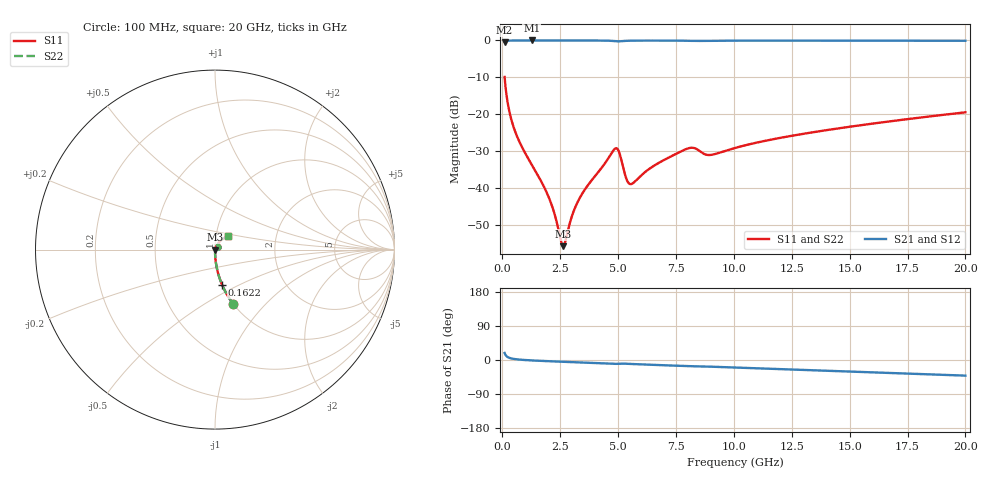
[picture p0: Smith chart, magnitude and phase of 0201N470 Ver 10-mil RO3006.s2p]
# GHz S MA R 50
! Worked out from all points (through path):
!   1601 points, 100 MHz to 20 GHz, reference 50 ohm
!   highest |S21| = -0.01 dB at 1.269 GHz (marker M1); lowest = -0.5 dB at 100 MHz (marker M2)
!   group delay of S21, straight-line fit = 5.97 ps
!   lowest |S11| = -55.8 dB at 2.625 GHz (marker M3), VSWR 1.00, Z = 50.2 - j0.0251 ohm
!   |S11| at or under -10 dB: 101.2 MHz to end of sweep
!   |S22| runs from -55.8 to -9.9 dB; largest |S21 - S12| = 0
!   S11 on the Smith chart (normalised r, x): 100 MHz: 1.00, -0.67; 162.2 MHz: 1.00, -0.41; 20 GHz: 1.14, +0.18
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0.1  0.3195 -71.5  0.9472 18.5  0.9472 18.5  0.3195 -71.5
0.1621875  0.2031 -78.4  0.9787 11.4  0.9787 11.4  0.2031 -78.4
0.3114375  0.1064 -84.2  0.9938 5.5  0.9938 5.5  0.1064 -84.2
0.522875  0.06203 -86.8  0.9975 2.6  0.9975 2.6  0.06203 -86.8
1.269125  0.02071 -88.3  0.9988 -1.1  0.9988 -1.1  0.02071 -88.3
2.04025  0.007008 -82.1  0.9986 -3.3  0.9986 -3.3  0.007008 -82.1
2.53775  0.001883 -37.9  0.9984 -4.5  0.9984 -4.5  0.001883 -37.9
2.624812  0.001617 -8.9  0.9983 -4.7  0.9983 -4.7  0.001617 -8.9
2.724312  0.001891 23.7  0.9983 -5.0  0.9983 -5.0  0.001891 23.7
3.085  0.004843 61.7  0.9981 -5.8  0.9981 -5.8  0.004843 61.7
3.420812  0.008032 68.3  0.9978 -6.6  0.9978 -6.6  0.008032 68.3
4.876  0.03416 38.1  0.9768 -10.2  0.9768 -10.2  0.03416 38.1
5.02525  0.03158 15.4  0.9712 -9.8  0.9712 -9.8  0.03158 15.4
5.348625  0.01354 8.5  0.987 -9.9  0.987 -9.9  0.01354 8.5
5.52275  0.01125 29.1  0.9911 -10.3  0.9911 -10.3  0.01125 29.1
6.741625  0.02166 65.2  0.9953 -13.3  0.9953 -13.3  0.02166 65.2
8.084875  0.0347 54.6  0.988 -16.4  0.988 -16.4  0.0347 54.6
8.930625  0.02787 50.9  0.9892 -17.5  0.9892 -17.5  0.02787 50.9
10.05  0.03475 61.4  0.9939 -19.9  0.9939 -19.9  0.03475 61.4
13.37081  0.05648 58.5  0.9936 -27.0  0.9936 -27.0  0.05648 58.5
16.69162  0.07947 52.4  0.9916 -34.1  0.9916 -34.1  0.07947 52.4
20  0.1059 45.9  0.9886 -41.2  0.9886 -41.2  0.1059 45.9
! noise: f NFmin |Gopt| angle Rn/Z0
0.1  0.000416  0.8986  0.2906  0.0008966
2.301  0.003649  0.7543  4.149  0.002995
4.515  0.0109  0.8317  8.092  0.0136
6.729  0.01067  0.7552  12.02  0.008716
8.943  0.01883  0.8104  15.97  0.0203
11.14  0.01416  0.7053  19.74  0.009166
13.36  0.01536  0.6807  23.52  0.008939
15.57  0.01698  0.6679  27.26  0.009295
17.79  0.01869  0.6592  30.96  0.009764
20  0.02043  0.6531  34.6  0.01026
